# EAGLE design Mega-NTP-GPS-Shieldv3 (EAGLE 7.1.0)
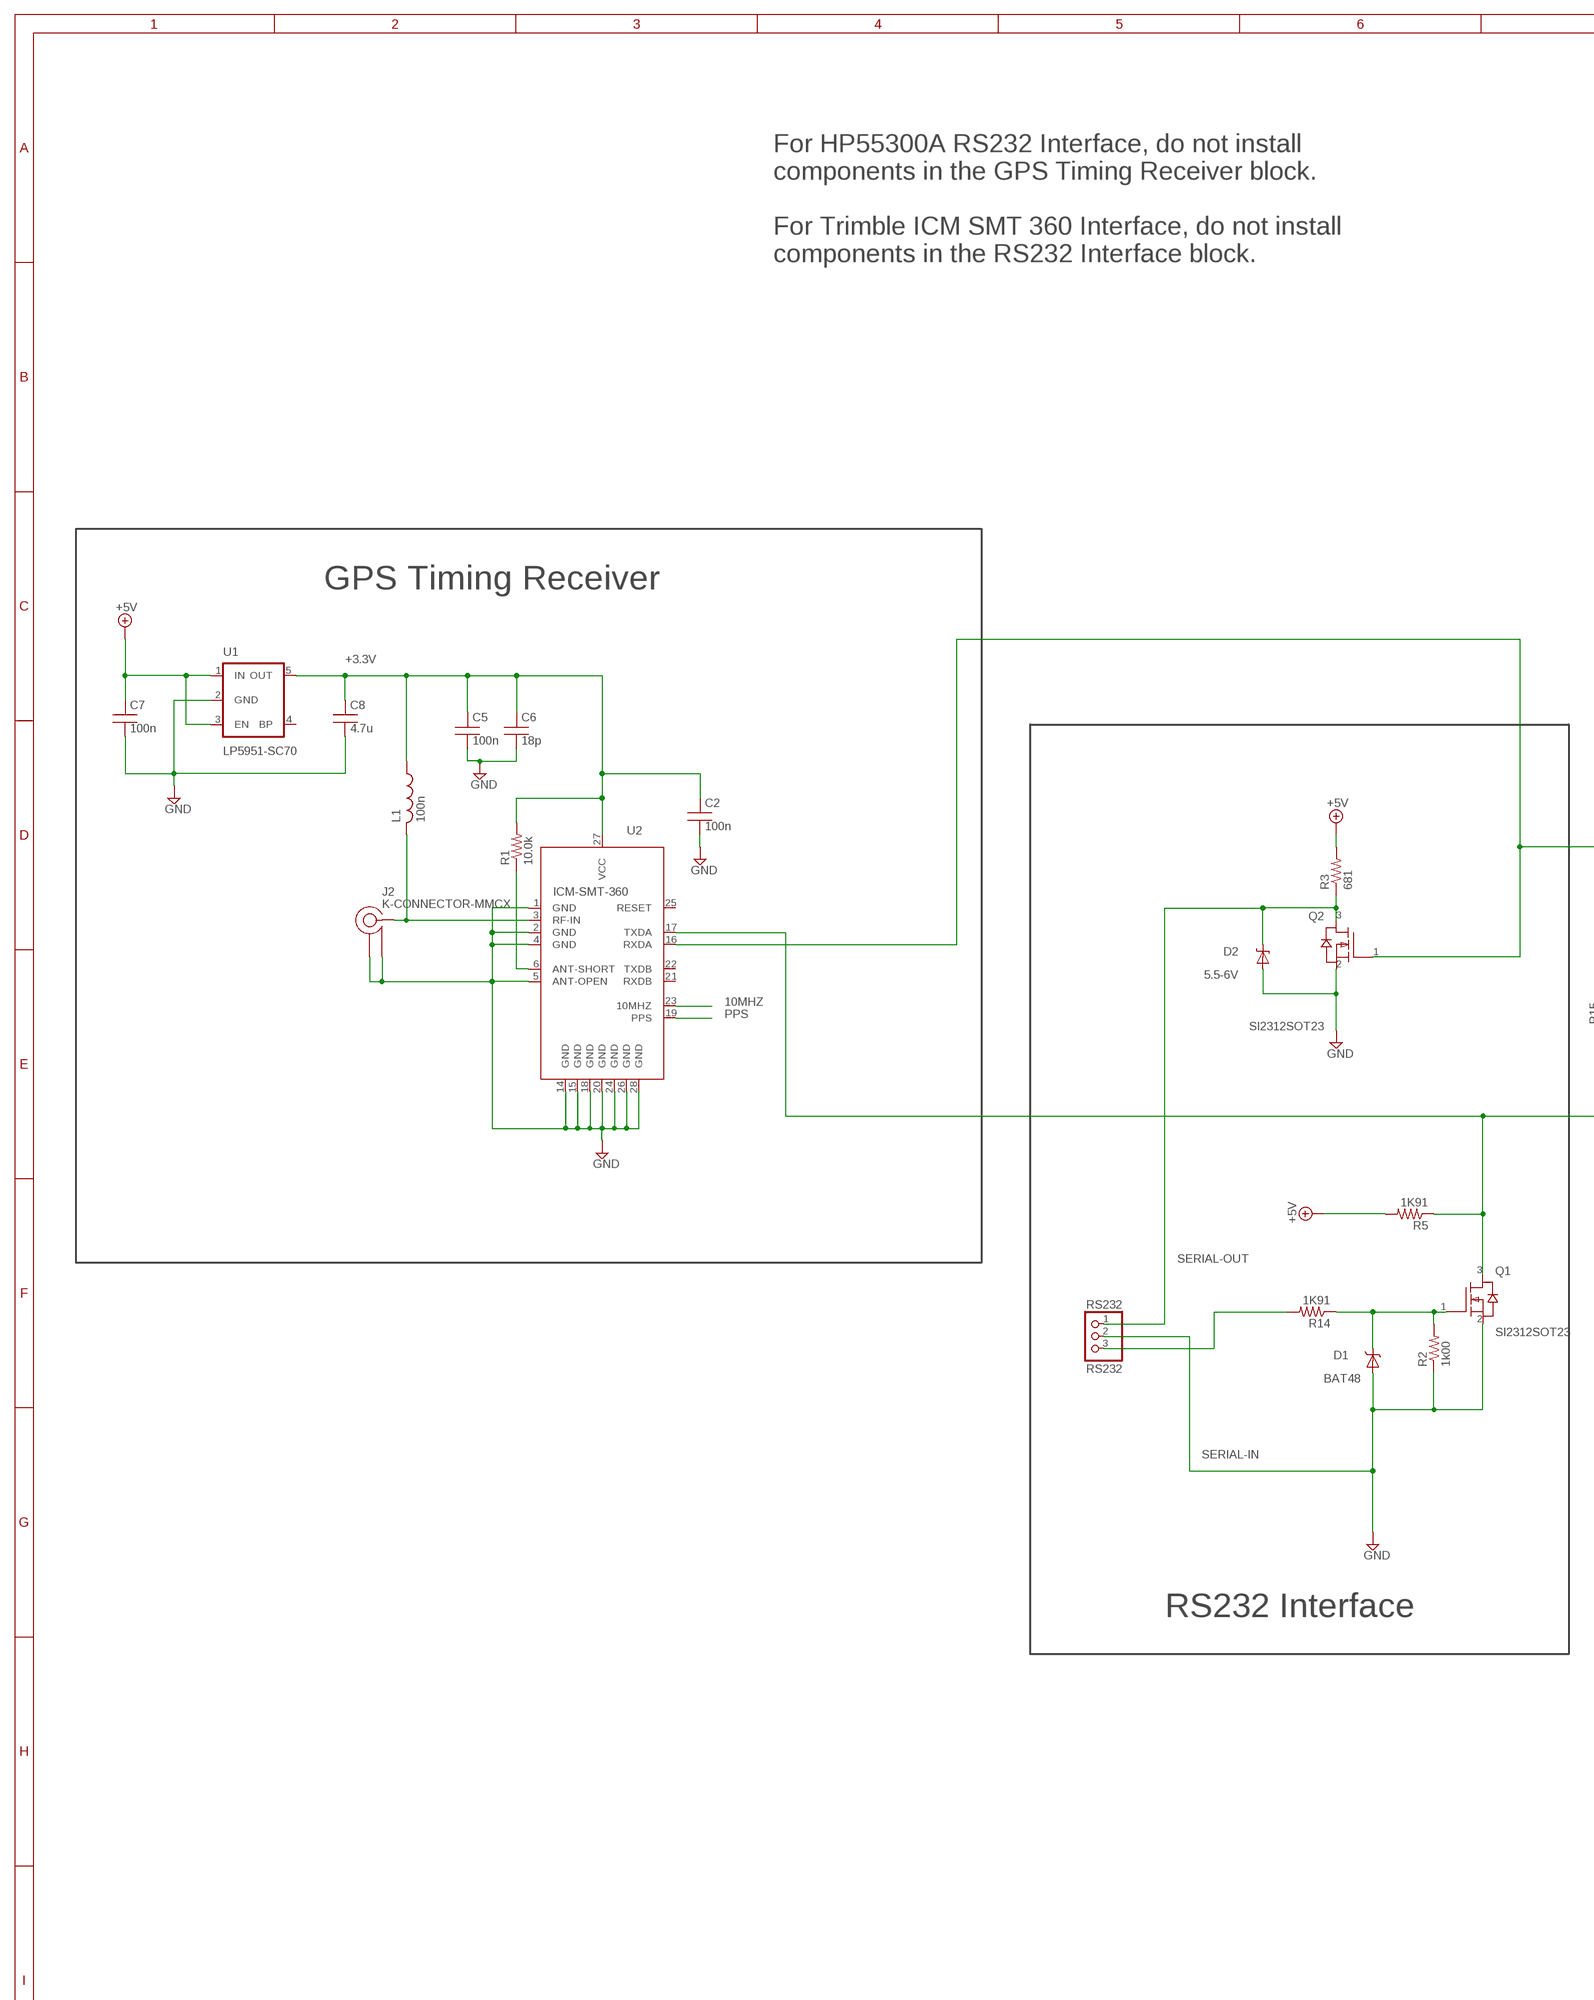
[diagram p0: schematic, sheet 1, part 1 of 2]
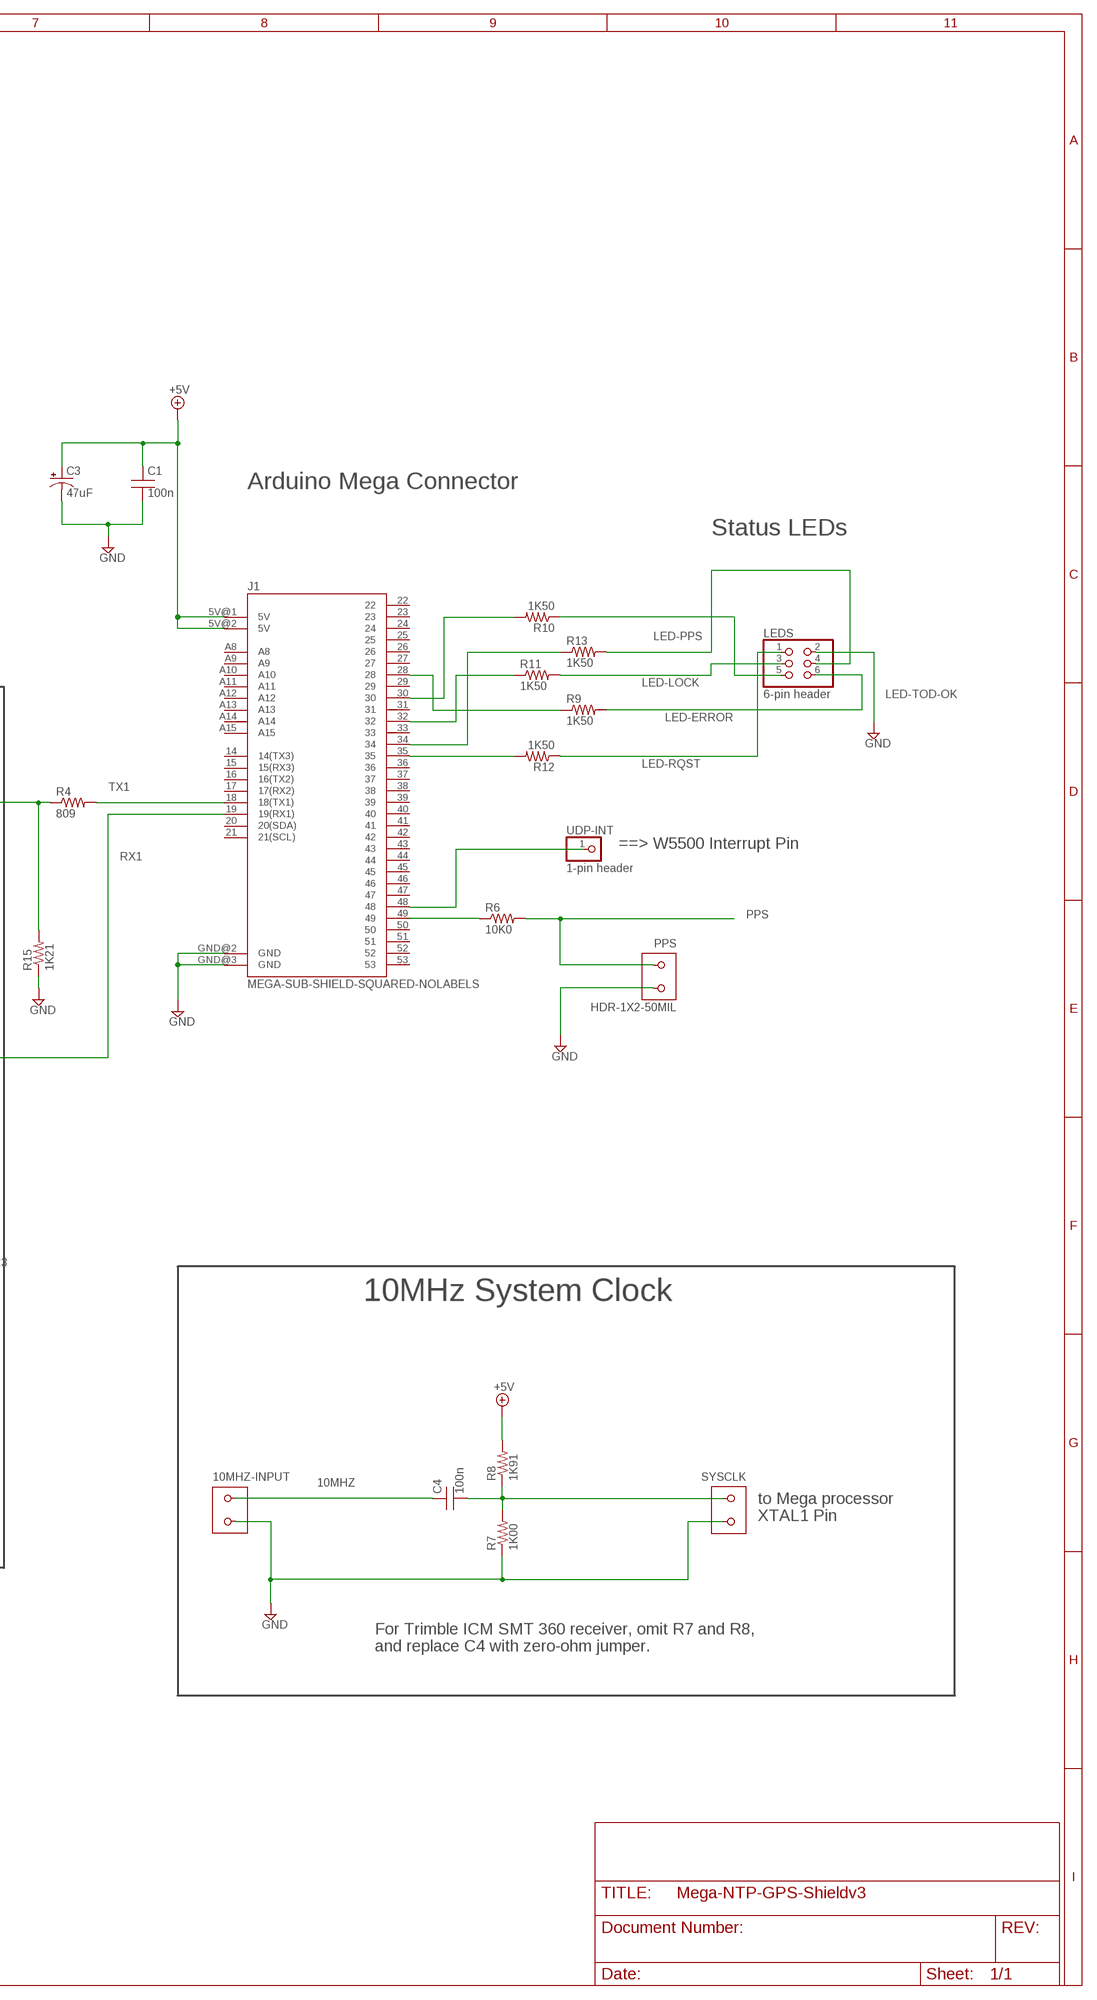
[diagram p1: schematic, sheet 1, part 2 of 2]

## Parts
10MHZ-INPUT  HDR-1X2-100MIL  [1X02-100MIL]
C1  100n  C-AVX-0805  [AVX-0805]
C2  100n  C-AVX-0805-NT  [AVX-0805-NT]
C3  47uF  47UF-TANT  [EIA3528]
C4  100n  C-AVX-0603  [AVX-0603]
C5  100n  C-AVX-0603-NT  [AVX-0603-NT]
C6  18p  C-AVX-0402-NT  [AVX-0402-NT]
C7  100n  C-AVX-0603-NT  [AVX-0603-NT]
C8  4.7u  C-AVX-0805-NT  [AVX-0805-NT]
D1  BAT48  DIODE-SCHOTTKY-SOD323  [SOD-323]
D2  5.5-6V  DIODE-ZENER-BZT52  [SOD-323]
J1  MEGA-SUB-SHIELD-SQUARED-NOLABELS  [MEGA-SUB-SHIELD-SQUARED-NOLABELS]
J2  K-CONNECTOR-MMCX  [MOLEX-MMCX-VERTICAL]
L1  100n  MURATA-LQW04A-LQW181-NT  [AVX-0603-NT]
LEDS  6-pin header  HDR-2X3-ROW-SWAP-50MIL  [2X03-50MIL]
PPS  HDR-1X2-50MIL  [1X02-50MIL]
Q1  SI2312SOT23  [SOT23]
Q2  SI2312SOT23  [SOT23]
R1  10.0k  R-AVX-0603  [AVX-0603]
R2  1k00  R-AVX-0603-NT  [AVX-0603-NT]
R3  681  R-AVX-0603  [AVX-0603]
R4  809  R-AVX-0603  [AVX-0603]
R5  1K91  R-AVX-0603  [AVX-0603]
R6  10K0  R-AVX-0603  [AVX-0603]
R7  1K00  R-AVX-0603  [AVX-0603]
R8  1K91  R-AVX-0603  [AVX-0603]
R9  1K50  R-AVX-0603  [AVX-0603]
R10  1K50  R-AVX-0603  [AVX-0603]
R11  1K50  R-AVX-0603  [AVX-0603]
R12  1K50  R-AVX-0603  [AVX-0603]
R13  1K50  R-AVX-0603  [AVX-0603]
R14  1K91  R-AVX-0603  [AVX-0603]
R15  1K21  R-AVX-0603-NT  [AVX-0603-NT]
RS232  RS232  HDR-1X3-ALL-SWAP-100-MIL  [1X03-100MIL]
SYSCLK  HDR-1X2-100MIL  [1X02-100MIL]
U1  LP5951-SC70  V_REG_LDOSMD2  [SC70]
U2  ICM-SMT-360  TRIMBLE-ICM-SMT-360-GPS-TIMING-MODULE  [TRIMBLE-ICM-SMT-360]
UDP-INT  1-pin header  PINHD-1X1  [1X01]

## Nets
10MHZ: 10MHZ-INPUT.1 C4.1 U2.23(10MHZ)
+3.3V: C2.1 C5.1 C6.1 C8.1 L1.1 R1.2 U1.5(OUT) U2.27(VCC)
+5V: C1.1 C3.A(+) C7.1 J1.5V@1(5V) J1.5V@2(5V) R3.2 R5.2 R8.2 U1.1(IN) U1.3(EN)
ANTENNA: J2.CENTER L1.2 U2.3(RF-IN)
GND: 10MHZ-INPUT.2 C1.2 C2.2 C3.C(-) C5.2 C6.2 C7.2 C8.2 D1.2(A) D2.2(A) J1.GND@2(GND) J1.GND@3(GND) J2.GND1 J2.GND2 LEDS.2 PPS.2 Q1.2(S) Q2.2(S) R2.1 R7.1 R15.1 RS232.2 SYSCLK.2 U1.2(GND) U2.1(GND) U2.2(GND) U2.4(GND) U2.5(ANT-OPEN) U2.14(GND) U2.15(GND) U2.18(GND) U2.20(GND) U2.24(GND) U2.26(GND) U2.28(GND)
LED-ERROR: LEDS.6 R9.2
LED-LOCK: LEDS.3 R11.2
LED-PPS: LEDS.4 R13.2
LED-RQST: LEDS.1 R12.1
LED-TOD-OK: LEDS.5 R10.1
N$1: Q2.1(G) R4.1 R15.2 U2.16(RXDA)
N$3: C4.2 R7.2 R8.1 SYSCLK.1
N$4: R1.1 U2.6(ANT-SHORT)
N$7: J1.49 R6.1
N$10: D1.1(C) Q1.1(G) R2.2 R14.1
N$11: J1.48 UDP-INT.1
N$17: J1.34 R13.1
N$18: J1.35 R12.2
N$19: J1.32 R11.1
N$20: J1.30 R10.2
N$21: J1.28 R9.1
PPS: PPS.1 R6.2 U2.19(PPS)
RX1: J1.19(19(RX1)) Q1.3(D) R5.1 U2.17(TXDA)
SERIAL-IN: R14.2 RS232.3
SERIAL-OUT: D2.1(C) Q2.3(D) R3.1 RS232.1
TX1: J1.18(18(TX1)) R4.2
Unconnected: J1.14(14(TX3)) J1.15(15(RX3)) J1.16(16(TX2)) J1.17(17(RX2)) J1.20(20(SDA)) J1.21(21(SCL)) J1.22 J1.23 J1.24 J1.25 J1.26 J1.27 J1.29 J1.31 J1.33 J1.36 J1.37 J1.38 J1.39 J1.40 J1.41 J1.42 J1.43 J1.44 J1.45 J1.46 J1.47 J1.50 J1.51 J1.52 J1.53 J1.A8 J1.A9 J1.A10 J1.A11 J1.A12 J1.A13 J1.A14 J1.A15 U1.4(BP) U2.21(RXDB) U2.22(TXDB) U2.25(RESET)

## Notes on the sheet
- For HP55300A RS232 Interface, do not install
  components in the GPS Timing Receiver block.
  
  For Trimble ICM SMT 360 Interface, do not install 
  components in the RS232 Interface block.
- Arduino Mega Connector
- Status LEDs
- GPS Timing Receiver
- ==> W5500 Interrupt Pin
- 10MHz System Clock
- to Mega processor
  XTAL1 Pin
- RS232 Interface
- For Trimble ICM SMT 360 receiver, omit R7 and R8,
  and replace C4 with zero-ohm jumper.

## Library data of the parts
10MHZ-INPUT PPS SYSCLK = max-local:HDR-1X2: Discrete wire thru-hole pattern (2-wires)
C1 C2 = max-local:C-AVX-0805: AVX 0805 SMT Capacitor; MFR: AVX; MPN: 0805(3/5)C104(J/K)ATxx
C3 = SparkFun-Capacitors:47UF-TANT: 47uF Tantalum SMT; MFR: Vishay/Sprague; MPN: TR3B476K010C0350; PROD_ID: CAP-08310
C4 C5 C7 = max-local:C-AVX-0603: AVX 0603 SMT Capacitor; MFR: AVX; MPN: 0603(3/5)C104(J/K)ATxx
C6 = max-local:C-AVX-0402; MFR: AVX; MPN: 04025A180JATxx
C8 = max-local:C-AVX-0805: AVX 0805 SMT Capacitor; MFR: AVX; MPN: C0805YC475KATxx
D1 = SparkFun-DiscreteSemi:DIODE-SCHOTTKY: Commonly MBRA140.
D2 = SparkFun-DiscreteSemi:DIODE-ZENER: Zener Diode
J1 = SparkFun-Boards:MEGA-SUB-SHIELD: Shield for Mega that only uses lower pins Will not interfere with shields like the Ethernet which need to plug into the ICSP pins.
J2 = max-local:K-CONNECTOR: K-Connector; DIGIKEY: WM3914CT-ND; MFR: Molex; MPN: 73415-206x
L1 = max-local:MURATA-LQW04A: Murata high-frequency wirewound SMT inductors; MFR: Murata; MPN: LQW18ANR10J00
LEDS = max-local:HDR-2X3-ROW-SWAP
Q1 Q2 = max-local:SI2312: Siliconix Si2313 N-channel MOSFET 20V, 6A, 0.026 ohm (4.5V Vgs); MFR: Siliconix; MPN: SI2312BDS
R1 = max-local:R-AVX-0603: SMT 0603 Resistor; MFR: Vishay/Dale; MPN: CRCW060310.0kFKxx
R2 R14 R15 = max-local:R-AVX-0603: SMT 0603 Resistor; MFR: Vishay/Dale; MPN: CRCW06034K02FKxx
R3 = max-local:R-AVX-0603: SMT 0603 Resistor; MFR: Vishay/Dale; MPN: CRCW0603DNP (681)FKxx
R4 R5 R7 R8 = max-local:R-AVX-0603: SMT 0603 Resistor; MFR: Vishay/Dale; MPN: CRCW06031K91FKxx
R6 = max-local:R-AVX-0603: SMT 0603 Resistor; MFR: Vishay/Dale; MPN: CRCW060310K0FKxx
R9-R13 = max-local:R-AVX-0603: SMT 0603 Resistor; MFR: Vishay/Dale; MPN: CRCW06031K50FKxx
RS232 = max-local:HDR-1X3-ALL-SWAP
U1 = SparkFun-PowerIC:V_REG_LDO: Voltage Regulator LDO Standard 150mA LDO voltage regulator in SOT-23 layout. Micrel part MIC5205. BP (by-pass) pin is used to lower output noise with 470pF cap.; MFR: TI; MPN: LP5951MG-3.3/NOPB
U2 = max-local:TRIMBLE-ICM-SMT-360-GPS-TIMING-MODULE: Trimble GPS Timing Module ICM 360 SMT; MFR: Trimble; MPN: ICM-SMT-360
UDP-INT = pinhead:PINHD-1X1: PIN HEADER

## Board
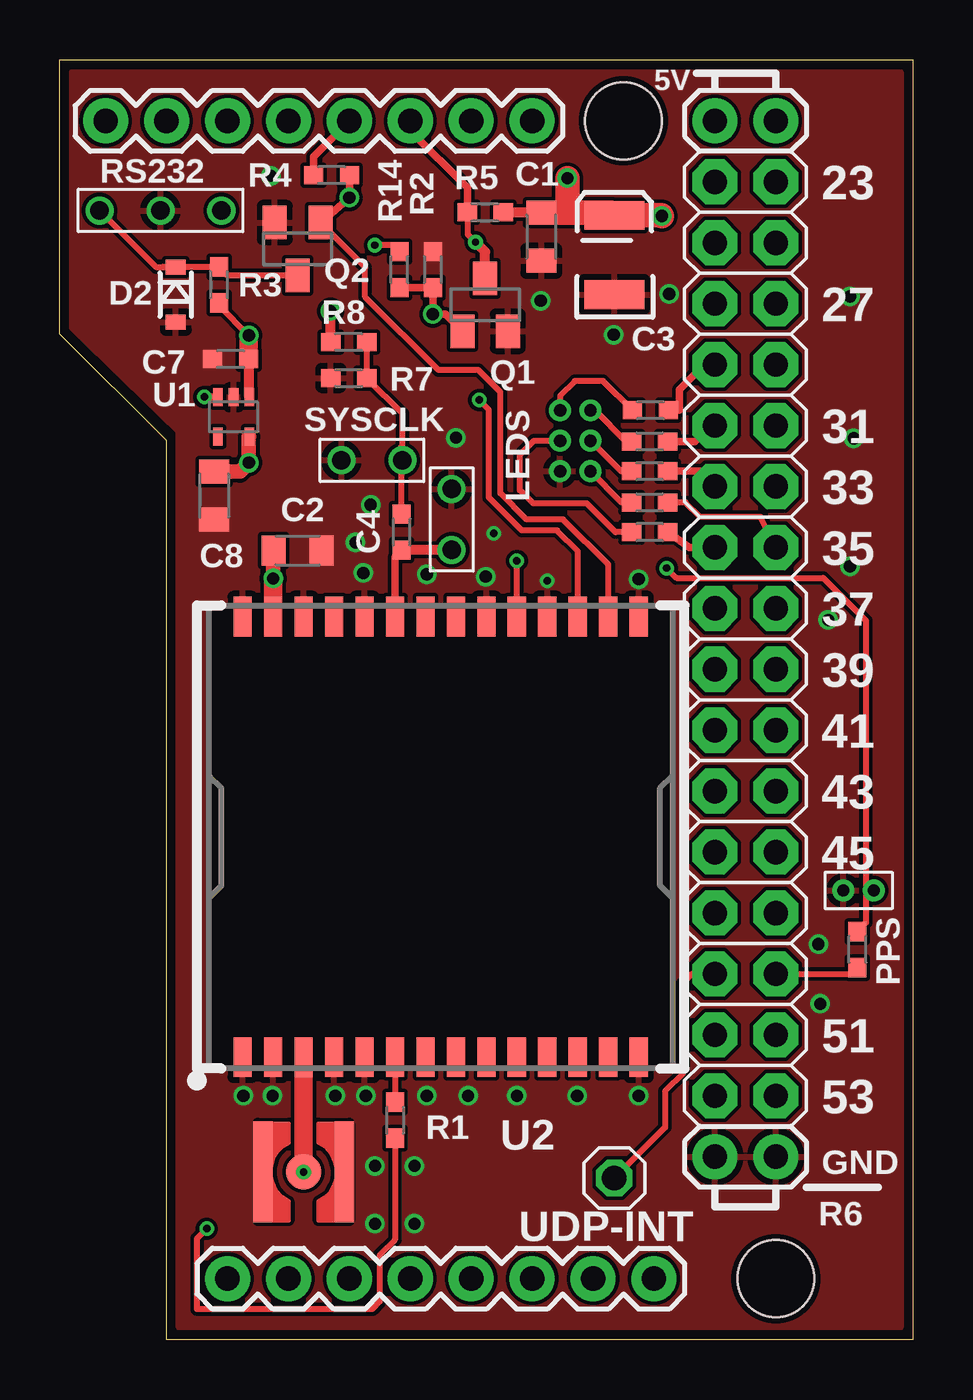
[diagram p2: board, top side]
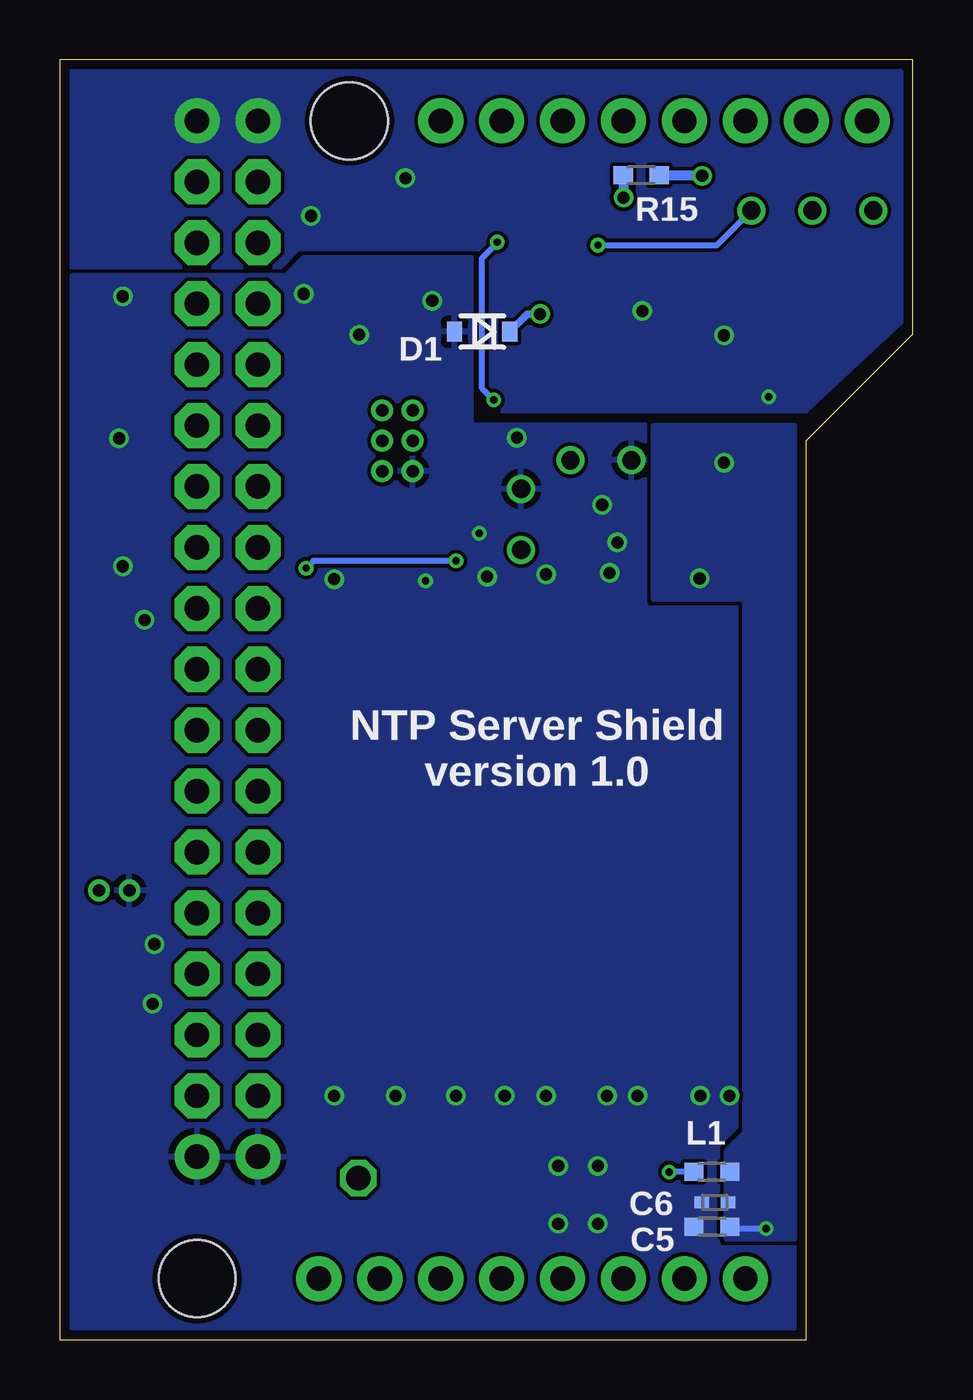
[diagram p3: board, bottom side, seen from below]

Size 35.56 x 53.34 mm. Coordinates in mm from the lower left corner, seen from the top.
Copper layers (1*16): Top 0.035mm / dielectric 1.5mm / Bottom 0.035mm
Design rules "SeeedStudio_2layer_DRU_no_angle_20140221 *": minimum track width 6mil, minimum drill 12mil, track to track 6mil, track to pad 6mil, pad to pad 6mil, via to via 6mil, smd to smd 0mil, copper to edge 10mil, drill to drill 10mil, minimum pad ring 8mil, minimum via ring 6mil, stop-mask expansion 2mil, vias tented up to drill 100mil, thermal gap 10mil

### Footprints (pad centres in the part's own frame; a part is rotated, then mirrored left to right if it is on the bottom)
1X02-100MIL = drill 0.762: 1 -1.27,0; 2 1.27,0
AVX-0805 = smd 1 x 1.25: 1 -1,0; 2 1,0
AVX-0805-NT = smd 1 x 1.25: 1 -1,0; 2 1,0
EIA3528 = smd 1.2 x 2.5: A 1.65,0; C -1.65,0
AVX-0603 = smd 0.8 x 0.75: 1 -0.75,0; 2 0.75,0
AVX-0603-NT = smd 0.8 x 0.75: 1 -0.75,0; 2 0.75,0
AVX-0402-NT = smd 0.6 x 0.5: 1 -0.55,0; 2 0.55,0
SOD-323 = smd 0.63 x 0.83: 1 -1.15,0; 2 1.15,0
MEGA-SUB-SHIELD-SQUARED-NOLABELS = drill 1.016 pad 1.88: 5V@1 27.305,50.8; 5V@2 29.845,50.8; 14 1.905,50.8; 15 4.445,50.8; 16 6.985,50.8; 17 9.525,50.8; 18 12.065,50.8; 19 14.605,50.8; 20 17.145,50.8; 21 19.685,50.8; A8 6.985,2.54; A9 9.525,2.54; A10 12.065,2.54; A11 14.605,2.54; A12 17.145,2.54; A13 19.685,2.54; A14 22.225,2.54; A15 24.765,2.54; GND@2 27.305,7.62; GND@3 29.845,7.62 | drill 1.016 pad 1.88 octagon: 22 27.305,48.26; 23 29.845,48.26; 24 27.305,45.72; 25 29.845,45.72; 26 27.305,43.18; 27 29.845,43.18; 28 27.305,40.64; 29 29.845,40.64; 30 27.305,38.1; 31 29.845,38.1; 32 27.305,35.56; 33 29.845,35.56; 34 27.305,33.02; 35 29.845,33.02; 36 27.305,30.48; 37 29.845,30.48; 38 27.305,27.94; 39 29.845,27.94; 40 27.305,25.4; 41 29.845,25.4; 42 27.305,22.86; 43 29.845,22.86; 44 27.305,20.32; 45 29.845,20.32; 46 27.305,17.78; 47 29.845,17.78; 48 27.305,15.24; 49 29.845,15.24; 50 27.305,12.7; 51 29.845,12.7; 52 27.305,10.16; 53 29.845,10.16 | hole 3.2: 23.495,50.8; 29.845,2.54
MOLEX-MMCX-VERTICAL = smd 1.473 x 1.473: CENTER 0,0 | smd 0.813 x 4.216: GND1 -1.702,0; GND2 1.702,0
2X03-50MIL = drill 0.508 pad 0.914: 1 -1.27,-0.635; 2 -1.27,0.635; 3 0,-0.635; 4 0,0.635; 5 1.27,-0.635; 6 1.27,0.635
1X02-50MIL = drill 0.508: 1 -0.635,0; 2 0.635,0
SOT23 = smd 1 x 1.4: 1 -0.95,-1.1; 2 0.95,-1.1; 3 0,1.1
1X03-100MIL = drill 0.762: 1 -2.54,0; 2 0,0; 3 2.54,0
SC70 = smd 0.4 x 0.75: 1 -0.65,-0.825; 2 0,-0.825; 3 0.65,-0.825; 4 0.65,0.825; 5 -0.65,0.825
TRIMBLE-ICM-SMT-360 = smd 1.651 x 0.762: 1 -9.182,8.255; 2 -9.182,6.985; 3 -9.182,5.715; 4 -9.182,4.445; 5 -9.182,3.175; 6 -9.182,1.905; 7 -9.182,0.635; 8 -9.182,-0.635; 9 -9.182,-1.905; 10 -9.182,-3.175; 11 -9.182,-4.445; 12 -9.182,-5.715; 13 -9.182,-6.985; 14 -9.182,-8.255; 15 9.182,-8.255; 16 9.182,-6.985; 17 9.182,-5.715; 18 9.182,-4.445; 19 9.182,-3.175; 20 9.182,-1.905; 21 9.182,-0.635; 22 9.182,0.635; 23 9.182,1.905; 24 9.182,3.175; 25 9.182,4.445; 26 9.182,5.715; 27 9.182,6.985; 28 9.182,8.255
1X01 = drill 1.016 octagon: 1 0,0

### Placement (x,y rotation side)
10MHZ-INPUT  16.33,34.19 90 top
C1  20.07,45.97 270 top
C2  9.91,32.89 0 top
C3  23.11,45.21 90 top
C4  14.25,33.66 90 top
C5  8.38,4.7 180 bottom
C6  8.26,5.71 180 bottom
C7  7.11,40.87 180 top
C8  6.43,35.18 270 top
D1  17.96,42.01 180 bottom
D2  4.83,43.56 270 top
J1  0,0 0 top
J2  10.16,6.99 0 top
L1  8.38,6.99 180 bottom
LEDS  21.49,37.47 90 top
PPS  33.3,18.72 180 top
Q1  17.73,43.13 0 top
Q2  9.91,45.47 180 top
R1  13.97,9.14 270 top
R2  15.54,44.6 270 top
R3  6.63,43.97 270 top
R4  11.33,48.54 180 top
R5  17.73,46.99 0 top
R6  33.25,16.26 90 top
R7  12.04,40.08 0 top
R8  12.04,41.58 180 top
R9  24.61,38.73 180 top
R10  24.59,37.44 0 top
R11  24.59,36.2 180 top
R12  24.59,34.9 0 top
R13  24.59,33.66 180 top
R14  14.15,44.6 90 top
R15  11.33,48.54 180 bottom
RS232  4.19,47.07 0 top
SYSCLK  13,36.65 180 top
U1  7.24,38.46 180 top
U2  15.88,20.95 90 top
UDP-INT  23.11,6.73 0 top

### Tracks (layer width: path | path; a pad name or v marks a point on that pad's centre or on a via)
10MHZ
  Top 0.305: U2.23 13.97,32.63 C4.1
  Top 0.406: 10MHZ-INPUT.1 C4.1
+3.3V  (via drill 0.3, 0.51)
  Top 0.254: R1.2 13.97,4.17 13.34,3.53 13.34,1.57 13.03,1.27 5.71,1.27 5.71,4.22 v6.12,4.62
  Top 0.61: U1.5 7.87,37.63 v7.87,36.55 7.5,36.18 C8.1 | v8.89,31.73 8.89,33.16 C2.1
  Top 0.762: U2.27 v8.89,31.73
  Bottom 0.254: v6.12,4.62 7.56,4.62 C5.1
  pour Bottom: 4.95,38.1 4.95,30.86 10.79,30.86 10.79,38.1
  pour Bottom: 4.95,30.99 4.95,4.19 7.75,4.19 7.75,7.87 6.99,8.64 6.99,30.99
+5V  (via drill 0.3, 0.51)
  Top 0.254: v7.87,41.86 6.63,43.1 R3.2
  Top 0.305: U1.3 5.91,39.28 v6.02,39.29
  Top 0.406: R5.2 20.05,46.99 C1.1 | U1.1 7.89,40.84 C7.1 | R8.2 11.29,42.86 v11.28,42.88
  Top 0.762: C7.1 7.86,41.85 v7.87,41.86
  Top 1.016: v25.09,46.84 25.07,46.86 C3.A 23,46.97 C1.1 | v21.16,48.41 21.16,46.99
  pour Bottom (rank 2, no thermals): 4.45,38.73 0.51,42.42 0.51,52.83 35.05,52.83 35.05,38.73
ANTENNA  (via drill 0.3)
  Top 0.762: U2.3 J2.CENTER
  Bottom 0.254: L1.2 J2.CENTER
  other vias: 10.16,6.99
GND  (via drill 0.3, 0.51)
  Bottom 0.406: R15.1 8.79,48.54 v8.79,48.51
  other vias: 12.32,33.22 17.75,31.8 18.08,33.6 20.32,31.62 24.13,10.16 31.62,16.48 31.7,14 32.03,30 32.94,32.23 17.02,10.16 15.29,10.16 19.05,10.16 21.56,10.16 11.48,10.16 8.86,10.16 7.65,10.16 33.1,37.57 15.29,31.9 16.51,37.59 12.95,34.8 32.94,43.48 25.4,43.59 20.04,43.31 12.65,31.95 13.13,7.24 13.13,4.83 14.78,4.83 14.78,7.24 12.75,10.16 23.09,41.88 24.13,31.7
  pour Top: 4.95,0.51 4.95,37.85 0.51,42.16 0.51,52.83 35.05,52.83 35.05,0.51
  pour Bottom (rank 2): 4.95,38.1 35.05,38.1 35.05,0.51 4.95,0.51
  pour Bottom: 18.41,36.2 18.41,45.09 25.4,45.09 26.14,44.32 35.05,44.32 35.05,36.2
LED-ERROR
  Top 0.254: R9.2 22.64,39.95 21.46,39.95 20.85,39.34 LEDS.6
LED-LOCK
  Top 0.254: R11.2 23.39,36.2 LEDS.3
LED-PPS
  Top 0.254: R13.2 23.16,33.66 21.97,34.85 19.74,34.85 19.18,35.41 19.18,36.88 19.76,37.47 LEDS.4
LED-RQST
  Top 0.254: R12.1 23.42,34.9 LEDS.1
LED-TOD-OK
  Top 0.254: R10.1 23.6,37.44 22.3,38.73
  Top 0.305: 22.3,38.73 LEDS.5
N$1  (via drill 0.51)
  Top 0.254: U2.16 22.86,32.31 20.98,34.19 19.46,34.19 18.36,35.28 18.36,39.5 17.45,40.41 15.77,40.41 12.72,43.46 12.72,44.7 Q2.1
  Top 0.305: R15.2 12.06,48.54 v12.06,47.6 Q2.1
  Bottom 0.406: R15.2 12.06,48.54 v12.06,47.6
N$3
  Top 0.254: R8.1 R7.2 14.28,38.6 SYSCLK.1 14.25,37.26 C4.2
N$4
  Top 0.254: U2.6 R1.1
N$7
  Top 0.254: J1.49 33.03,15.24 R6.1
N$10  (via drill 0.51)
  Top 0.305: R14.1 R2.2 v15.54,42.75 16.07,42.75 Q1.1
  Bottom 0.305: v15.54,42.75 16.07,42.75 D1.1
N$11
  Top 0.254: J1.48 26.34,15.24 25.98,14.88 25.98,11.12 25.22,10.36 25.22,8.84 UDP-INT.1
N$17
  Top 0.305: J1.34 26.25,33.02 R13.1
N$18
  Top 0.254: J1.35 29.21,34.29 26.7,34.29 26.09,34.9 R12.2
N$19
  Top 0.305: J1.32 26.67,36.2 R11.1
N$20
  Top 0.305: J1.30 26.47,37.44 R10.2
N$21
  Top 0.305: J1.28 26.87,40.64 25.83,39.6 25.83,38.75 R9.1
PPS  (via drill 0.3)
  Top 0.254: 33.6,18.75 33.6,29.97 31.83,31.75 25.7,31.75 v25.3,32.16 | 33.6,18.75 33.6,17.38 R6.2 | PPS.1 33.63,18.72 33.6,18.75 | U2.19 v19.05,32.46
  Bottom 0.254: v19.05,32.46 24.99,32.46 v25.3,32.16
RX1  (via drill 0.3)
  Top 0.254: U2.17 21.59,32.87 20.73,33.73 19.25,33.73 17.88,35.1 17.88,38.76 v17.48,39.17 | 16.99,47 16.99,46.91 16.99,46.08 v17.32,45.74
  Top 0.305: J1.19 14.61,50.39 16.99,48.01 16.99,47
  Top 0.406: v17.32,45.74 17.73,45.34 Q1.3 | R5.1 16.99,46.99 16.99,46.91
  Bottom 0.254: v17.48,39.17 17.96,39.65 17.96,45.09 17.32,45.72 v17.32,45.74
SERIAL-IN  (via drill 0.3)
  Top 0.254: R14.2 13.88,45.62 v13.13,45.62
  Bottom 0.254: v13.13,45.62 8.18,45.62 RS232.3
SERIAL-OUT
  Top 0.254: RS232.1 4.01,44.71 D2.1 4.27,44.72 R3.1 6.98,44.37 Q2.3
TX1
  Top 0.305: R4.2 10.58,49.31 J1.18

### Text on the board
bPlace: NTP Server Shield / version 1.0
